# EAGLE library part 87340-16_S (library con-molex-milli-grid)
RECEPTACAL
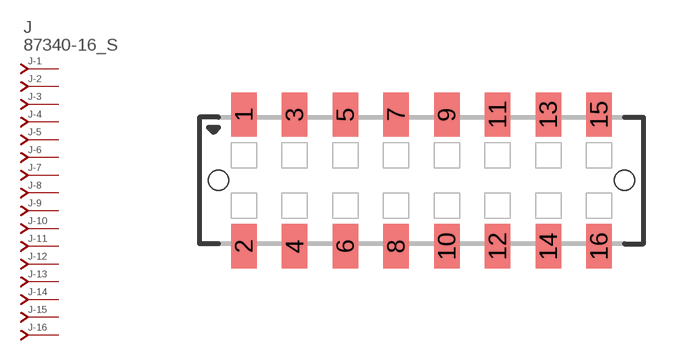
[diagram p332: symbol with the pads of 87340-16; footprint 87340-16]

Designator prefix J; gates -1=J-NV -2=J-N -3=J-N -4=J-N -5=J-N -6=J-N -7=J-N -8=J-N -9=J-N -10=J-N -11=J-N -12=J-N -13=J-N -14=J-N -15=J-N -16=J-N

## 87340-16_S  [87340-16]
1  -1:J  pas
2  -2:J  pas
3  -3:J  pas
4  -4:J  pas
5  -5:J  pas
6  -6:J  pas
7  -7:J  pas
8  -8:J  pas
9  -9:J  pas
10  -10:J  pas
11  -11:J  pas
12  -12:J  pas
13  -13:J  pas
14  -14:J  pas
15  -15:J  pas
16  -16:J  pas

## Footprint 87340-16 (pad centres in mm)
RECEPTACAL SMD Dual Row, Vertical, Low Profile
smd 1 x 1.75: 1 -7,2.6; 2 -7,-2.6; 3 -5,2.6; 4 -5,-2.6; 5 -3,2.6; 6 -3,-2.6; 7 -1,2.6; 8 -1,-2.6; 9 1,2.6; 10 1,-2.6; 11 3,2.6; 12 3,-2.6; 13 5,2.6; 14 5,-2.6; 15 7,2.6; 16 7,-2.6
hole 0.8 at -8,0
hole 0.8 at 8,0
